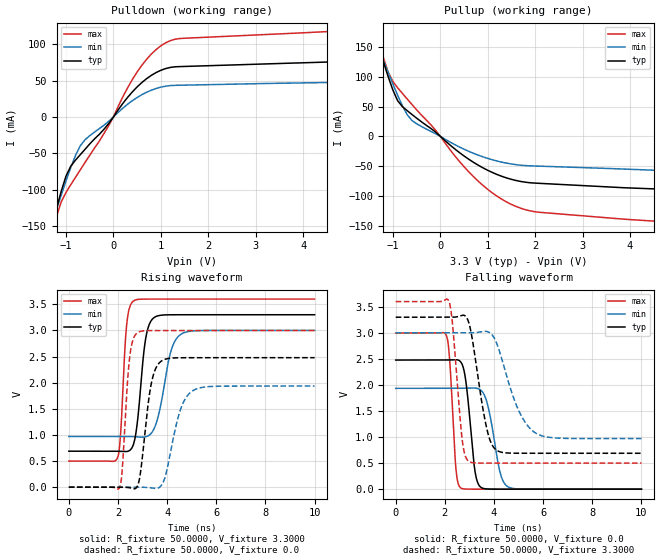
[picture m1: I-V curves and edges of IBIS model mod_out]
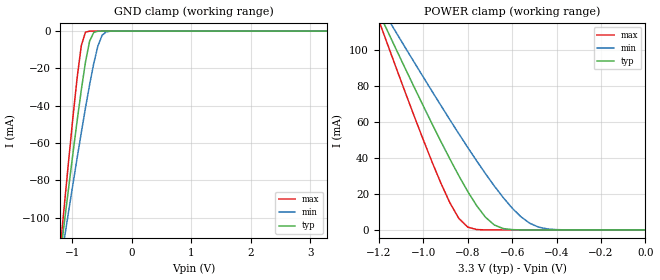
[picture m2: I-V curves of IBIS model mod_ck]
| IBIS (I/O, Buffer, Information, Specification) Model, officially
| electronic behavioral standard for Buffer structures of digital pins.
[IBIS ver]  4.0
[File name] rhfac2525_3v3.ibs
[File Rev]  1.0
[Date]   19 Oct 2023
[Source]   CAD & Design Services (Catania) - STMicroelectronics
[Notes]
   (Note1)  This IBIS model includes the 14L ceramic package data
   (Note2)  This IBIS model has some Notes about the non-monotonicity
   of the I-V curves, but they are not indicative of problems
   inside the model;
[Copyright] (c) 2023 STMicroelectronics
|   Component RHFAC2525
[Component] RHFAC2525
[Manufacturer] STMicroelectronics
[Package]
| variable   typ   min   max
R_pkg   0.0   0.0   0.0
L_pkg   0.0H   0.0H   0.0H
C_pkg   0.0F   0.0F   0.0F
[Pin]  signal_name   model_name   R_pin   L_pin   C_pin
1   O0   mod_out   83.7m   2.67nH   1.03pF
2   O2   mod_out   28.3m   0.78nH   1.07pF
3   NC   NC   34.9m   0.88nH   0.82pF
4   GND   GND   34.9m   0.88nH   0.82pF
5   VCC   POWER   34.9m   0.88nH   0.82pF
6   O4   mod_out   28.3m   0.78nH   1.07pF
7   O6   mod_out   83.7m   2.67nH   1.03pF
8   O7   mod_out   83.7m   2.67nH   1.03pF
9   O5   mod_out   28.3m   0.78nH   1.07pF
10   GND   GND   34.9m   0.88nH   0.82pF
11   VCC   POWER   34.9m   0.88nH   0.82pF
12   CKIN   mod_ck   34.9m   0.88nH   0.82pF
13   O3   mod_out   28.3m   0.78nH   1.07pF
14   O1   mod_out   83.7m   2.67nH   1.03pF
| Models and submodels in the file (2): mod_out (Output), mod_ck (Input)
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|   Model mod_out
[Model]   mod_out
Model_type Output
|Vinl  =   0.660V
|Vinh  =   2.640V
Vmeas  =   1.650V
Cref   =   50pF
Rref   =   500
C_comp   11.120pF   10.610pF   11.610pF
[Temperature Range]  25.0000   0.1250k   -55.0000
[Voltage Range]   3.3000V   3.0000V   3.6000V
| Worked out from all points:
|   slope of the pulldown table from 0 to 0.495 V, typ, clamps not added: 12.1 ohm
|   slope of the pullup table from 0 to 0.495 V, typ, clamps not added: 15.1 ohm
|   rising waveform, R_fixture 50.0000, V_fixture 3.3000: 20-80 % time 324ps typ, 502ps min, 208ps max; typ from 0.689 V to 3.3 V
|   rising waveform, R_fixture 50.0000, V_fixture 0.0: 20-80 % time 382ps typ, 575ps min, 244ps max; typ from 0 V to 2.48 V
|   falling waveform, R_fixture 50.0000, V_fixture 0.0: 20-80 % time 305ps typ, 437ps min, 209ps max; typ from 2.48 V to 0 V
|   falling waveform, R_fixture 50.0000, V_fixture 3.3000: 20-80 % time 531ps typ, 890ps min, 318ps max; typ from 3.3 V to 0.689 V
[Pulldown]
|Voltage   I(typ)   I(min)   I(max)
-3.3V     -694.6mA   -572.3mA   -860mA
-1.4V     -176.9mA   -168.2mA   -195.6mA
-1.3V     -151.1mA   -147.7mA   -164.6mA
-1.1V     -102.2mA   -107.5mA   -116.8mA
-1V       -81.56mA   -88.11mA   -103.9mA
-800mV    -59.46mA   -52.96mA   -83.2mA
-600mV    -44.64mA   -31.5mA    -62.76mA
-100mV    -9.051mA   -6.066mA   -11.96mA
500mV     41.4mA     26.84mA    62mA
800mV     57.35mA    36.89mA    86.71mA
1.2V      68.23mA    43.22mA    105.1mA
6.6V      79.81mA    49.5mA     123.9mA
[Pullup]
|Voltage   I(typ)   I(min)   I(max)
-3.3V     695.4mA    573.2mA    860.6mA
-1.5V     203.4mA    189.5mA    227.7mA
-1.4V     176.9mA    168.7mA    194.4mA
-1.1V     100.5mA    107.6mA    108mA
-900mV    59.91mA    69.03mA    81.67mA
-700mV    43.29mA    36.6mA     62.96mA
-600mV    36.9mA     26.78mA    53.78mA
700mV     -43.72mA   -28.56mA   -67.87mA
1.2V      -64.28mA   -41.62mA   -100.9mA
1.6V      -74.32mA   -47.66mA   -118mA
2.1V      -79.08mA   -50.15mA   -127.8mA
6.6V      -95.03mA   -63.23mA   -153mA
[Ramp]
| variable   typ   min   max
dV/dt_r   1.4866/0.4160n   1.1609/0.5991n   1.7990/0.2714n
dV/dt_f   1.5662/0.5475n   1.2177/0.9284n   1.8602/0.3525n
R_load = 50.0000
[Rising Waveform]
R_fixture= 50.0000
V_fixture= 3.3000
V_fixture_min= 3.0000
V_fixture_max= 3.6000
|time   V(typ)   V(min)   V(max)
0s        688.9mV    970.8mV    500mV
2.01ns    687mV      971.2mV    599.7mV
2.11ns    684.4mV    971.3mV    1.04V
2.35ns    681.6mV    970.8mV    3.091V
2.63ns    816mV      966.8mV    3.564V
3.11ns    2.794V     963mV      3.6V
3.45ns    3.239V     1.101V     3.6V
4.17ns    3.299V     2.626V     3.6V
4.59ns    3.3V       2.934V     3.6V
10ns      3.3V       3V         3.6V
[Rising Waveform]
R_fixture= 50.0000
V_fixture= 0.0
V_fixture_min= 0.0
V_fixture_max= 0.0
|time   V(typ)   V(min)   V(max)
0s        127pV      40.18nV    92.94pV
2.06ns    742.2uV    -5.772uV   -17.73mV
2.18ns    558.8uV    46.43uV    373.6mV
2.48ns    -11.32mV   338.4uV    2.5V
2.8ns     31.05mV    619.1uV    2.959V
3.34ns    1.944V     -12.55mV   2.997V
3.78ns    2.418V     43.33mV    2.997V
4.5ns     2.476V     1.423V     2.997V
5.04ns    2.478V     1.844V     2.997V
10ns      2.478V     1.935V     2.997V
[Falling Waveform]
R_fixture= 50.0000
V_fixture= 0.0
V_fixture_min= 0.0
V_fixture_max= 0.0
|time   V(typ)   V(min)   V(max)
0s        2.478V     1.935V     2.997V
2.07ns    2.478V     1.935V     2.942V
2.21ns    2.48V      1.935V     2.388V
2.45ns    2.485V     1.935V     396.9mV
2.67ns    2.426V     1.936V     17.08mV
2.87ns    2.016V     1.939V     1.527mV
3.23ns    335mV      1.941V     95.88uV
3.45ns    42.01mV    1.905V     22.4uV
4.55ns    48.94uV    51.25mV    -126.4nV
10ns      -1.68nV    33.13nV    -143.7nV
[Falling Waveform]
R_fixture= 50.0000
V_fixture= 3.3000
V_fixture_min= 3.0000
V_fixture_max= 3.6000
|time   V(typ)   V(min)   V(max)
0s        3.3V       3V         3.6V
2.16ns    3.299V     3V         3.612V
2.32ns    3.3V       3V         3.132V
2.7ns     3.337V     2.999V     973.5mV
2.98ns    3.189V     2.999V     532.1mV
3.68ns    1.218V     3.029V     500.2mV
4.08ns    756.3mV    2.834V     500mV
4.92ns    689.9mV    1.601V     500mV
5.64ns    689mV      1.094V     500mV
10ns      688.9mV    970.8mV    500mV
|   Model mod_ck
[Model]   mod_ck
Model_type Input
Vinl  =   0.660V
Vinh  =   2.640V
C_comp   2.119pF   2.068pF   2.200pF
[Model Spec]
|hysteresis   (deltaV = 50mV)
Vinh+   1.680V   NA   NA
Vinh-   1.670V   NA   NA
Vinl+   1.630V   NA   NA
Vinl-   1.620V   NA   NA
[Temperature Range]  25.0000   0.1250k   -55.0000
[Voltage Range]   3.3000V   3.0000V   3.6000V
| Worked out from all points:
|   GND clamp passes 1 mA (typ) near -0.64 V on its own axis
|   POWER clamp passes 1 mA (typ) near -0.64 V on its own axis
[GND_clamp]
|Voltage   I(typ)   I(min)   I(max)
-3.3V     -693.7mA   -571.7mA   -857.3mA
-1.2V     -119.8mA   -124.6mA   -115.4mA
-1.13V    -101.4mA   -110.3mA   -91.83mA
-1.06V    -83.29mA   -96.03mA   -68.62mA
-920mV    -48.13mA   -68.05mA   -25.09mA
-850mV    -31.61mA   -54.45mA   -7.844mA
-780mV    -16.68mA   -41.25mA   -576.7uA
-710mV    -5.36mA    -28.7mA    -15.45uA
-640mV    -695uA     -17.26mA   -374.1nA
-500mV    -3.363uA   -2.228mA   -227.3pA
-430mV    -220.7nA   -380.2uA   -14.19pA
3.28V     6.534pA    5.68uA     5.92pA
[POWER_clamp]
|Voltage   I(typ)   I(min)   I(max)
-3.28V    689.2mA    568.4mA    851.1mA
-1.2V     120.7mA    125.6mA    116.3mA
-1.16V    110.2mA    117.4mA    102.8mA
-1.12V    99.73mA    109.2mA    89.34mA
-920mV    48.98mA    68.97mA    25.82mA
-840mV    30.13mA    53.42mA    6.464mA
-800mV    21.42mA    45.84mA    1.601mA
-720mV    7.079mA    31.25mA    29.17uA
-680mV    2.751mA    24.39mA    3.489uA
-520mV    8.135uA    3.699mA    711.4pA
-400mV    76.29nA    182.7uA    9.986pA
0V        6.622pA    2.268nA    7.2pA
